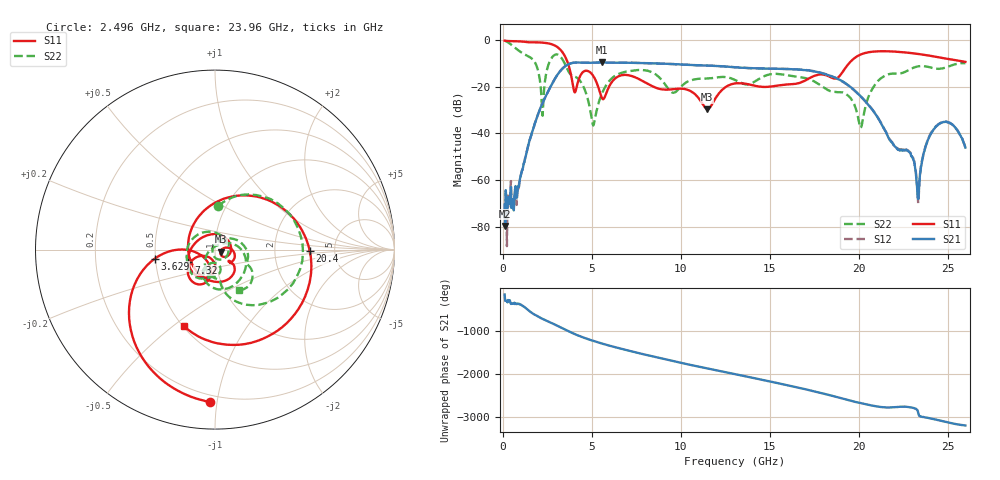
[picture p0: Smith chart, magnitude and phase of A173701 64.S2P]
!  2-Port S-parameters saved by WinCal
! VAR MeasName=S-Parameters (CALIBRATED_DATA) read from VNA (N5245A)
! VAR MeasDate=2017-6-7 10:32:41
! VAR NAME=A173701 64
! VAR FILENAME=A173701 64.S2P
! VAR DATE=2017-6-7 10:32:41
! VAR PHYS_PORTS=1,2
# Hz S DB R 50
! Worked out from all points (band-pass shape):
!   801 points, 100 MHz to 26 GHz, reference 50 ohm
!   highest |S21| = -9.65 dB at 5.571 GHz (marker M1); lowest = -79.6 dB at 132.4 MHz (marker M2)
!   |S21| within 3 dB of the highest: 3.305 GHz to 16.59 GHz (13.29 GHz wide, 134 % of centre); 16.63065 GHz to 16.6491 GHz (18.45 MHz wide, 0.111 % of centre)
!   lowest |S11| = -29.7 dB at 11.5 GHz (marker M3), VSWR 1.07, Z = 53.2 - j1.17 ohm
!   |S11| at or under -10 dB: 3.658 GHz to 19.46 GHz (15.8 GHz wide, 137 % of centre)
!   |S22| runs from -37.6 to -0.2 dB; largest |S21 - S12| = 0.0041
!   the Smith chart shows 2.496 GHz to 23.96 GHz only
!   S11 on the Smith chart (normalised r, x): 2.496 GHz: 0.16, -0.95; 3.629 GHz: 0.49, -0.06; 7.32 GHz: 0.73, -0.11; 20.4 GHz: 3.24, -0.09; 23.96 GHz: 0.51, -0.55
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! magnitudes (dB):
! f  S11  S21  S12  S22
! 100 MHz  -0.3  -70.5  -74.5  -0.2
! 132.4 MHz  -0.4  -79.6  -71.9  -0.4
! 1.751 GHz  -1.0  -37.0  -37.0  -9.0
! 2.204 GHz  -1.2  -27.5  -27.4  -29.6
! 2.496 GHz  -1.4  -22.8  -22.8  -12.3
! 3.629 GHz  -9.4  -10.7  -10.6  -12.6
! 4.05 GHz  -22.5  -9.7  -9.7  -15.7
! 4.438 GHz  -14.3  -9.8  -9.7  -18.7
! 5.086 GHz  -15.5  -9.7  -9.7  -36.6
! 5.571 GHz  -24.9  -9.6  -9.7  -23.0
! 7.32 GHz  -15.7  -9.8  -9.8  -13.1
! 8.744 GHz  -20.8  -10.1  -10.1  -15.7
! 11.5 GHz  -29.7  -11.0  -11.0  -16.5
! 13.05 GHz  -18.6  -11.7  -11.7  -17.2
! 17.39 GHz  -15.8  -13.4  -13.2  -17.4
! 20.11 GHz  -6.3  -24.1  -24.1  -37.6
! 20.4 GHz  -5.5  -26.5  -26.5  -28.1
! 21.69 GHz  -4.9  -42.1  -42.0  -14.7
! 23.35 GHz  -6.0  -68.0  -69.9  -11.3
! 23.96 GHz  -6.7  -41.7  -41.5  -11.6
! 24.96 GHz  -8.1  -35.2  -35.0  -11.6
! 26 GHz  -9.4  -46.1  -46.1  -10.0
